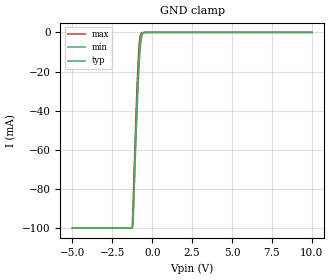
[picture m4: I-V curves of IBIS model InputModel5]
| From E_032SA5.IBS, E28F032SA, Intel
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|*************************Input Model 5****************************
[Model]   InputModel5
Model_type   Input
|   For CE#1
Vinl = 0.8V
Vinh = 2.0V
| Variable   typ   min   max
C_comp   5.61p   NA   7.6p
[Voltage Range]   5.0V   4.5V   5.5V
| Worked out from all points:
|   GND clamp passes 1 mA (typ) near -0.67 V on its own axis
[GND_clamp]
|Voltage I(typ)   I(min)   I(max)
-5V       -100mA     -100mA     -100mA
-1.25V    -100mA     -100mA     -100mA
-1.2V     -96.23mA   -97.79mA   -88.15mA
-1V       -46.56mA   -50.74mA   -38.9mA
-900mV    -25.12mA   -30.11mA   -18.44mA
-850mV    -16.38mA   -21.53mA   -10.56mA
-800mV    -9.116mA   -13.84mA   -4.805mA
-750mV    -4.18mA    -8.061mA   -1.736mA
-700mV    -1.581mA   -4.079mA   -585.7uA
-600mV    -227.3uA   -715.1uA   -151uA
-250mV    0A         0A         0A
10V       0A         0A         0A
[POWER_clamp]
| Input buffer circuits of this product do not intrinsically
| require a [POWER_clamp] definition.  This zero current
| [POWER_clamp] is provided for compatibility with some ibis
| parsers.
|   Voltage  I(typ)   I(min)   I(max)
-5V       0A         0A         0A
-4.75V    0A         0A         0A
9.75V     0A         0A         0A
10V       0A         0A         0A
